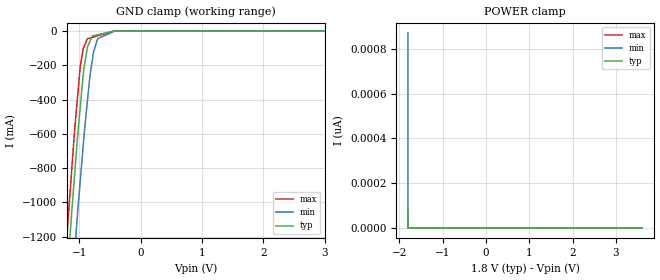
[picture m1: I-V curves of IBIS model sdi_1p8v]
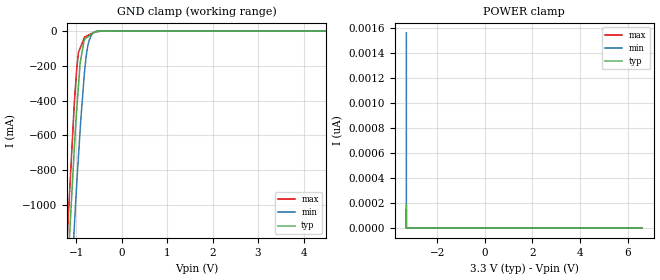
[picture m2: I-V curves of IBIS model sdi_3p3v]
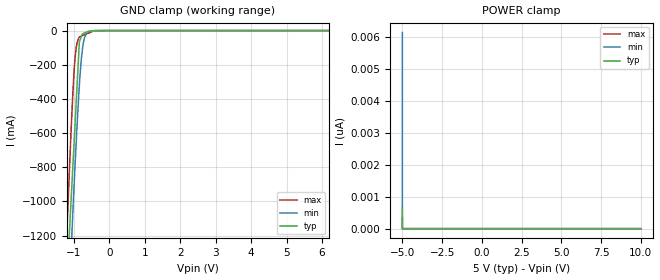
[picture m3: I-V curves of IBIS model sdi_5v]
|Texas Instruments Incorporated
| Marketing Part # : ADS127L11
| Digital Voltage Range : 1.65V-5.5V
| Package-type: QFN-RUK  / TSSOP -PW
| #pins/pkg drawing : QFN-20 RUK / TSSOP-20 PW
[IBIS Ver] 3.2
[File name] ads127l11.ibs
[File Rev] 1.0
[Date] 08/12/2021
[Source]
| Texas Instruments Incorporated.
| 12500 TI Blvd
| Dallas, TX -75243
[Notes] Revision History:
| Rev 1.0: 02/18/2019
| - Initial version of the model
| - Model generated from simulations in TISPICE/SPECTRE
| - C_comp although listed in numerical order of value are
| obtained from varying PVT conditions. For PVT conditions for
| each specific value refer the buffer description under
| respective [Model]. IBIS model user is responsible for using
| appropriate C_comp to simulate for Signal Integrity.
| - Warnings regarding combined Non-monotonicity of various models have been
| reviewed and considered minor and can be ignored.
|**** Modify the following if you use [Model Selector]*****************
| - Model names with a trailing _1p8v contain the model for 1.8V operation.
| - Model names with a trailing _3p3v contain the model for 3.3V operation.
| - Model names with a trailing _5v contain the model for 5V operation.
|- Model names with a _hp_ contain the model for half power / drive strength
|  operation.
|- Model names with a _fp_ contain the model for full power / drive strength
|  operation.
[Disclaimer]
| This model is designed as an aid for customers of Texas Instruments.
| TI and its licensors and suppliers make no warranties, either expressed
| or implied, with respect to this model, including the warranties of
| merchantability or fitness for a particular purpose. The model is
| provided solely on an "as is" basis. The entire risk as to its quality
| and performance is with the customer.
| This model is subject to change without notice. Texas Instruments
| Incorporated is not responsible for updating this model.
[Copyright]
(C) Copyright 2021 Texas Instruments Incorporated. All rights reserved.
| Component1 ADS127L11RUK (per package)
[Component] ADS127L11RUK
[Manufacturer] Texas Instruments Incorporated
[Package] |20 WQFN - RUK package
|variable typ min max
R_pkg 0.05 0.04 0.06
L_pkg 1.0nH 0.8nH 1.2nH
C_pkg 0.2pF 0.16pF 0.24pF
| pin number (pin name) mapping to model name
[Pin] signal_name   model_name   R_pin   L_pin   C_pin
1   AINP   NC   NA   NA   NA
2   AINN   NC   NA   NA   NA
3   VCM   NC   NA   NA   NA
4   REFP   NC   NA   NA   NA
5   REFN   NC   NA   NA   NA
6   RESETn   input_resetn   NA   NA   NA
7   CSn   input_sdi   NA   NA   NA
8   SDI   input_sdi   NA   NA   NA
9   SCLK   input_sdi   NA   NA   NA
10   SDO/DRDYn   output   NA   NA   NA
11   DRDYn   output   NA   NA   NA
12   CLK   input_sdi   NA   NA   NA
13   IOVDD   NC   NA   NA   NA
14   DGND   NC   NA   NA   NA
15   CAPD   NC   NA   NA   NA
16   START   input_start   NA   NA   NA
17   AVSS   NC   NA   NA   NA
18   CAPA   NC   NA   NA   NA
19   AVDD2   NC   NA   NA   NA
20   AVDD1   NC   NA   NA   NA
|***** end of component 1 definition
| Component1 ADS127L11PW (per package)
[Component] ADS127L11PW
[Manufacturer] Texas Instruments Incorporated
[Package] |20 TSSOP - PW package
|variable typ min max
R_pkg 0.05 0.04 0.06
L_pkg 1.0nH 0.8nH 1.2nH
C_pkg 0.2pF 0.16pF 0.24pF
| pin number (pin name) mapping to model name
[Pin] signal_name   model_name   R_pin   L_pin   C_pin
1   CAPA   NC   NA   NA   NA
2   AVDD2   NC   NA   NA   NA
3   AVDD1   NC   NA   NA   NA
4   AINP   NC   NA   NA   NA
5   AINN   NC   NA   NA   NA
6   VCM   NC   NA   NA   NA
7   REFP   NC   NA   NA   NA
8   REFN   NC   NA   NA   NA
9   RESETn   input_resetn   NA   NA   NA
10   CSn   input_sdi   NA   NA   NA
11   SDI   input_sdi   NA   NA   NA
12   SCLK   input_sdi   NA   NA   NA
13   SDO/DRDYn   output   NA   NA   NA
14   DRDYn   output   NA   NA   NA
15   CLK   input_sdi   NA   NA   NA
16   IOVDD   NC   NA   NA   NA
17   DGND   NC   NA   NA   NA
18   CAPD   NC   NA   NA   NA
19   START   input_start   NA   NA   NA
20   AVSS   NC   NA   NA   NA
|***** end of component 2 definition
|***Modify the following as it applies to a speciic model with multiple ****
|*** powver supply options or driver programmability *********
[Model Selector] input_sdi
sdi_1p8v input buffer at 1.8V operation.
sdi_3p3v input buffer at 3.3V operation.
sdi_5v input buffer at 5.0V operation.
[Model Selector] input_resetn
resetn_1p8v input buffer at 1.8V operation.
resetn_3p3v input buffer at 3.3V operation.
resetn_5v input buffer at 5.0V operation.
[Model Selector] input_start
start_1p8v input buffer at 1.8V operation.
start_3p3v input buffer at 3.3V operation.
start_5v input buffer at 5.0V operation.
[Model Selector] output
drdyn_fp_1p8v output buffer at 1.8V operation with full power/drive strength.
drdyn_fp_3p3v output buffer at 3.3V operation with full power/drive strength.
drdyn_fp_5v output buffer at 5.0V operation with full power/drive strength.
drdyn_hp_1p8v output buffer at 1.8V operation with half power/drive strength.
drdyn_hp_3p3v output buffer at 3.3V operation with half power/drive strength.
drdyn_hp_5v output buffer at 5.0V operation with half power/drive strength.
| Models and submodels in the file (15): sdi_1p8v (Input), sdi_3p3v (Input), sdi_5v (Input), resetn_1p8v (Input), resetn_3p3v (Input), resetn_5v (Input), start_1p8v (Input), start_3p3v (Input), start_5v (Input), drdyn_fp_1p8v (3-state), drdyn_fp_3p3v (3-state), drdyn_fp_5v (3-state), drdyn_hp_1p8v (3-state), drdyn_hp_3p3v (3-state), drdyn_hp_5v (3-state)
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|   sdi_1p8v Model
[Model]   sdi_1p8v
Model_type   Input
Vinl = 0.54
Vinh = 1.26
|   typ   min   max
C_comp   0.6369pF   0.6369pF   0.6369pF
[Voltage Range]   1.8   1.65   1.95
[Temperature Range]   25   125   -40
[Power Clamp Reference]   1.8   1.65   1.95
[GND Clamp Reference]   0   0   0
[GND Clamp]
|   Voltage   I(typ)   I(min)   I(max)
-1.8V     -4.323A    -4.211A    -4.387A
-1.221V   -1.55A     -1.992A    -1.295A
-1.157V   -1.221A    -1.684A    -971.3mA
-1.079V   -848.8mA   -1.307A    -588.5mA
-1.028V   -613.5mA   -1.061A    -380.9mA
-985.1mV  -444.8mA   -875.7mA   -209.8mA
-936.5mV  -254.7mA   -666.1mA   -102.8mA
-869.6mV  -96.71mA   -414mA     -45.39mA
-766.2mV  -26.83mA   -119.7mA   -34.5mA
-702.3mV  -21.57mA   -44.93mA   -27.77mA
-425.9mV  -130.3uA   -130.6uA   -182.3uA
3.6V      0A         0A         0A
[POWER Clamp]
|   Voltage   I(typ)   I(min)   I(max)
-1.8V     89.43pA    870.7pA    72.46pA
-1.8V     0A         0A         0A
-1.8V     0A         0A         0A
3.6V      0A         0A         0A
|   sdi_3p3v Model
[Model]   sdi_3p3v
Model_type   Input
Vinl = 0.99
Vinh = 2.31
|   typ   min   max
C_comp   0.6369pF   0.6369pF   0.6369pF
[Voltage Range]   3.3   3   3.6
[Temperature Range]   25   125   -40
[Power Clamp Reference]   3.3   3   3.6
[GND Clamp Reference]   0   0   0
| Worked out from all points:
|   GND clamp passes 1 mA (typ) near -0.50 V on its own axis
[GND Clamp]
|   Voltage   I(typ)   I(min)   I(max)
-3.3V     -8.287A    -7.976A    -8.613A
-1.192V   -1.391A    -1.857A    -1.159A
-1.046V   -702.1mA   -1.155A    -441.8mA
-987.4mV  -450.7mA   -879.8mA   -216.7mA
-947.9mV  -309.6mA   -714.8mA   -120.7mA
-912.8mV  -183.8mA   -569.9mA   -98.05mA
-821.2mV  -47.93mA   -248.2mA   -39.09mA
-799.4mV  -43.94mA   -189.7mA   -31.84mA
-767.9mV  -38.16mA   -122.7mA   -27.84mA
-714.7mV  -28.42mA   -54.52mA   -21.1mA
-592.9mV  -6.137mA   -4.628mA   -6.366mA
6.6V      0A         0A         0A
[POWER Clamp]
|   Voltage   I(typ)   I(min)   I(max)
-3.3V     196pA      1.56nA     146.3pA
-3.3V     0A         0A         0A
-3.3V     0A         0A         0A
6.6V      0A         0A         0A
|   sdi_5v Model
[Model]   sdi_5v
Model_type   Input
Vinl = 1.5
Vinh = 3.5
|   typ   min   max
C_comp   0.6369pF   0.6369pF   0.6369pF
[Voltage Range]   5   4.5   5.5
[Temperature Range]   25   125   -40
[Power Clamp Reference]   5   4.5   5.5
[GND Clamp Reference]   0   0   0
[GND Clamp]
|   Voltage   I(typ)   I(min)   I(max)
-5V       -12.75A    -12.24A    -13.3A
-1.196V   -1.46A     -1.853A    -1.172A
-1.093V   -1.05A     -1.359A    -654.8mA
-1.066V   -942.4mA   -1.235A    -527.2mA
-1.031V   -803.8mA   -1.074A    -375.6mA
-962.2mV  -532.3mA   -773mA     -149.1mA
-914.1mV  -341.1mA   -571.8mA   -76.96mA
-844.9mV  -66.52mA   -320mA     -38.43mA
-795mV    -38.56mA   -179.1mA   -32.51mA
-734.7mV  -17.31mA   -74.31mA   -27.32mA
-557.7mV  -2.094mA   -6.268mA   -12.1mA
10V       0A         0A         0A
[POWER Clamp]
|   Voltage   I(typ)   I(min)   I(max)
-5V       649.3pA    6.158nA    353.7pA
-5V       0A         0A         0A
-5V       0A         0A         0A
10V       0A         0A         0A
